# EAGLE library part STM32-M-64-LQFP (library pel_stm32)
STM32F103 Medium Density 64pin LQFP
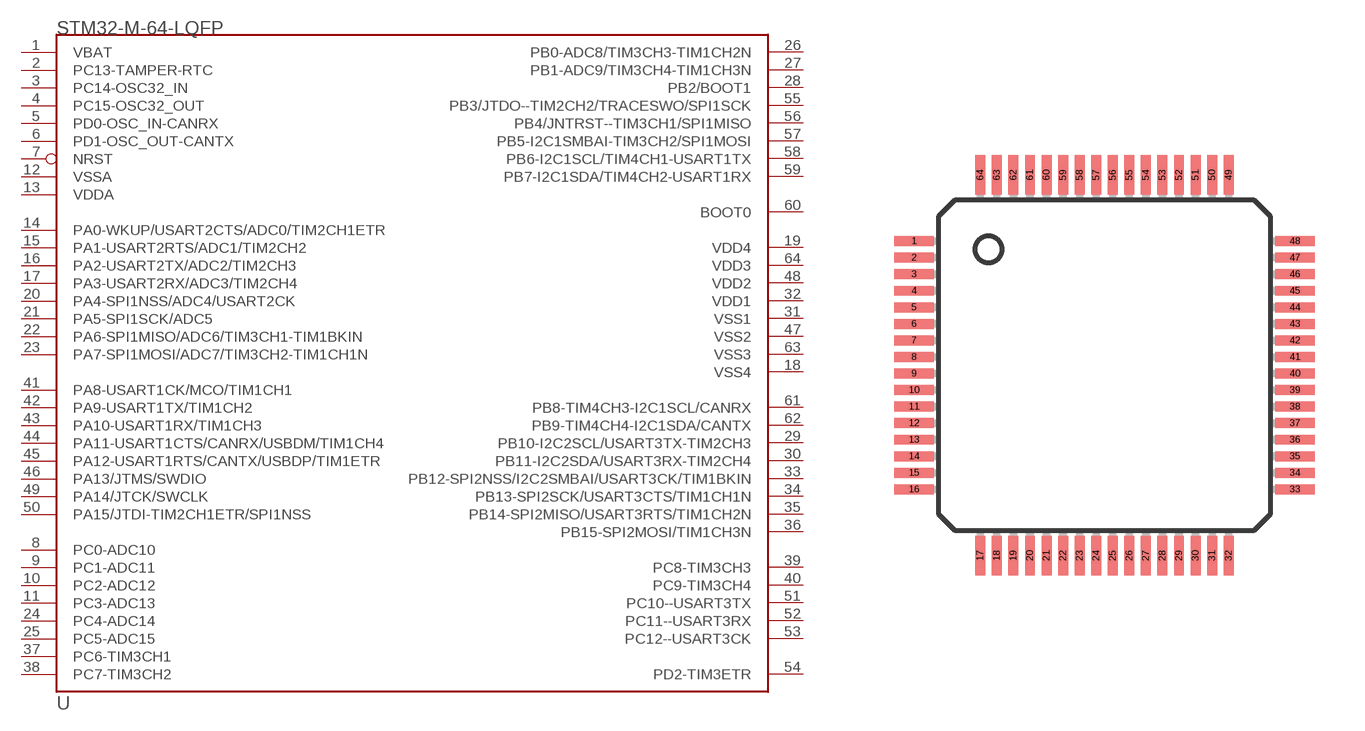
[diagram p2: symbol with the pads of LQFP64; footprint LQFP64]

Designator prefix U

## STM32-M-64-LQFP  [LQFP64]
1  VBAT  sup
2  PC13-TAMPER-RTC
3  PC14-OSC32_IN
4  PC15-OSC32_OUT
5  PD0-OSC_IN-CANRX  in
6  PD1-OSC_OUT-CANTX  out
7  NRST
8  PC0-ADC10
9  PC1-ADC11
10  PC2-ADC12
11  PC3-ADC13
12  VSSA  sup
13  VDDA  sup
14  PA0-WKUP/USART2CTS/ADC0/TIM2CH1ETR
15  PA1-USART2RTS/ADC1/TIM2CH2
16  PA2-USART2TX/ADC2/TIM2CH3
17  PA3-USART2RX/ADC3/TIM2CH4
18  VSS4
19  VDD4
20  PA4-SPI1NSS/ADC4/USART2CK
21  PA5-SPI1SCK/ADC5
22  PA6-SPI1MISO/ADC6/TIM3CH1-TIM1BKIN
23  PA7-SPI1MOSI/ADC7/TIM3CH2-TIM1CH1N
24  PC4-ADC14
25  PC5-ADC15
26  PB0-ADC8/TIM3CH3-TIM1CH2N
27  PB1-ADC9/TIM3CH4-TIM1CH3N
28  PB2/BOOT1
29  PB10-I2C2SCL/USART3TX-TIM2CH3
30  PB11-I2C2SDA/USART3RX-TIM2CH4
31  VSS1  sup
32  VDD1  sup
33  PB12-SPI2NSS/I2C2SMBAI/USART3CK/TIM1BKIN
34  PB13-SPI2SCK/USART3CTS/TIM1CH1N
35  PB14-SPI2MISO/USART3RTS/TIM1CH2N
36  PB15-SPI2MOSI/TIM1CH3N
37  PC6-TIM3CH1
38  PC7-TIM3CH2
39  PC8-TIM3CH3
40  PC9-TIM3CH4
41  PA8-USART1CK/MCO/TIM1CH1
42  PA9-USART1TX/TIM1CH2
43  PA10-USART1RX/TIM1CH3
44  PA11-USART1CTS/CANRX/USBDM/TIM1CH4
45  PA12-USART1RTS/CANTX/USBDP/TIM1ETR
46  PA13/JTMS/SWDIO
47  VSS2  sup
48  VDD2  sup
49  PA14/JTCK/SWCLK
50  PA15/JTDI-TIM2CH1ETR/SPI1NSS
51  PC10--USART3TX
52  PC11--USART3RX
53  PC12--USART3CK
54  PD2-TIM3ETR
55  PB3/JTDO--TIM2CH2/TRACESWO/SPI1SCK
56  PB4/JNTRST--TIM3CH1/SPI1MISO
57  PB5-I2C1SMBAI-TIM3CH2/SPI1MOSI
58  PB6-I2C1SCL/TIM4CH1-USART1TX
59  PB7-I2C1SDA/TIM4CH2-USART1RX
60  BOOT0  in
61  PB8-TIM4CH3-I2C1SCL/CANRX
62  PB9-TIM4CH4-I2C1SDA/CANTX
63  VSS3  sup
64  VDD3  sup

## Footprint LQFP64 (pad centres in mm)
Based on STM PCB landpattern recomendation
smd 1.2 x 0.3: 1 -5.75,3.75; 2 -5.75,3.25; 3 -5.75,2.75; 4 -5.75,2.25; 5 -5.75,1.75; 6 -5.75,1.25; 7 -5.75,0.75; 8 -5.75,0.25; 9 -5.75,-0.25; 10 -5.75,-0.75; 11 -5.75,-1.25; 12 -5.75,-1.75; 13 -5.75,-2.25; 14 -5.75,-2.75; 15 -5.75,-3.25; 16 -5.75,-3.75; 33 5.75,-3.75; 34 5.75,-3.25; 35 5.75,-2.75; 36 5.75,-2.25; 37 5.75,-1.75; 38 5.75,-1.25; 39 5.75,-0.75; 40 5.75,-0.25; 41 5.75,0.25; 42 5.75,0.75; 43 5.75,1.25; 44 5.75,1.75; 45 5.75,2.25; 46 5.75,2.75; 47 5.75,3.25; 48 5.75,3.75
smd 0.3 x 1.2: 17 -3.75,-5.75; 18 -3.25,-5.75; 19 -2.75,-5.75; 20 -2.25,-5.75; 21 -1.75,-5.75; 22 -1.25,-5.75; 23 -0.75,-5.75; 24 -0.25,-5.75; 25 0.25,-5.75; 26 0.75,-5.75; 27 1.25,-5.75; 28 1.75,-5.75; 29 2.25,-5.75; 30 2.75,-5.75; 31 3.25,-5.75; 32 3.75,-5.75; 49 3.75,5.75; 50 3.25,5.75; 51 2.75,5.75; 52 2.25,5.75; 53 1.75,5.75; 54 1.25,5.75; 55 0.75,5.75; 56 0.25,5.75; 57 -0.25,5.75; 58 -0.75,5.75; 59 -1.25,5.75; 60 -1.75,5.75; 61 -2.25,5.75; 62 -2.75,5.75; 63 -3.25,5.75; 64 -3.75,5.75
